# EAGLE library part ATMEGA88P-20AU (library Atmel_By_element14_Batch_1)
8-bit Microcontroller with 4/8/16/32K Bytes In-System Programmable Flash
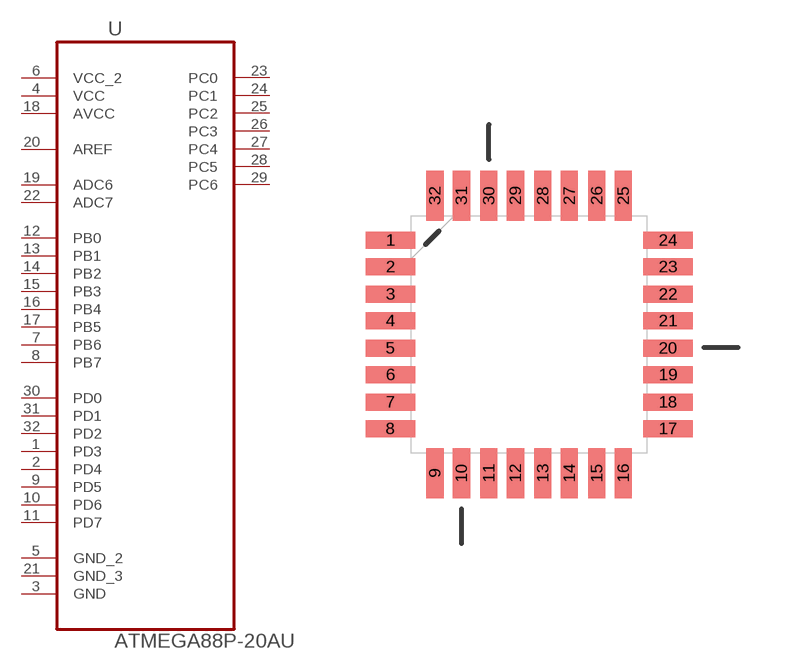
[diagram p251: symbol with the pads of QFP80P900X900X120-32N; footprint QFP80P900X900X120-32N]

Designator prefix U

## ATMEGA88P-20AU (MPN: ATMEGA88P-20AU; OC_FARNELL: 1636946; OC_NEWARK: 03P2032; PACKAGE: TQFP-32; SUPPLIER: ATMEL)  [QFP80P900X900X120-32N]
1  PD3
2  PD4
3  GND  pas
4  VCC  pwr
5  GND_2  pas
6  VCC_2  pwr
7  PB6
8  PB7
9  PD5
10  PD6
11  PD7
12  PB0
13  PB1
14  PB2
15  PB3
16  PB4
17  PB5
18  AVCC  pwr
19  ADC6  in
20  AREF  in
21  GND_3  pas
22  ADC7  in
23  PC0
24  PC1
25  PC2
26  PC3
27  PC4
28  PC5
29  PC6
30  PD0
31  PD1
32  PD2

## Footprint QFP80P900X900X120-32N (pad centres in mm)
smd 1.473 x 0.508: 1 -4.115,2.794; 2 -4.115,2.007; 3 -4.115,1.194; 4 -4.115,0.406; 5 -4.115,-0.406; 6 -4.115,-1.194; 7 -4.115,-2.007; 8 -4.115,-2.794; 17 4.115,-2.794; 18 4.115,-2.007; 19 4.115,-1.194; 20 4.115,-0.406; 21 4.115,0.406; 22 4.115,1.194; 23 4.115,2.007; 24 4.115,2.794
smd 0.508 x 1.473: 9 -2.794,-4.115; 10 -2.007,-4.115; 11 -1.194,-4.115; 12 -0.406,-4.115; 13 0.406,-4.115; 14 1.194,-4.115; 15 2.007,-4.115; 16 2.794,-4.115; 25 2.794,4.115; 26 2.007,4.115; 27 1.194,4.115; 28 0.406,4.115; 29 -0.406,4.115; 30 -1.194,4.115; 31 -2.007,4.115; 32 -2.794,4.115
